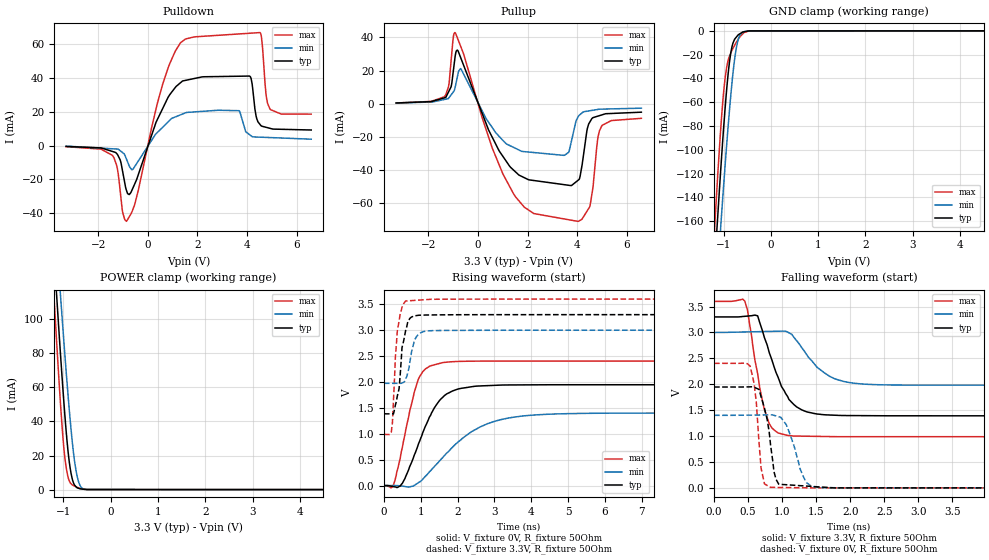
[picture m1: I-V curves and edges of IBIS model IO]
| Texas Instruments Incorporated
| UCD90120A 12-Rail Power Supply Sequencer and Monitor With ACPI Support
[IBIS ver]   4.1
[File name]   ucd90120a.ibs
[File Rev]   1.0
[Date]   02/22/2018
[Source]
| Texas Instruments Incorporated.
| Analog-eLab Design Center, HPA
| 12500 TI Blvd
| Dallas, TX -75243
[Notes]   Revision History:
| Rev 1.0: 02/22/2018
| - Initial version of the model
| - Model based on simulations from Spectre
| - Model not matched to measurements
| - C_comp although listed in numerical order of value are
|   obtained from varying PVT conditions. For PVT conditions for
|   each specific value refer the buffer description under
|   respective [Model]. IBIS model user is responsible for using
|   appropriate C_comp to simulate for Signal Integrity.
| - Warnings regarding combined Non-monotonicity of various models
|   have been reviewed and considered minor and can be ignored.
[Disclaimer]
| This model is designed as an aid for customers of Texas Instruments.
| TI and its licensors and suppliers make no warranties, either expressed
| or implied, with respect to this  model, including the warranties of
| merchantability or fitness for a particular purpose. The model is
| provided solely on an "as is" basis. The entire risk as to its quality
| and performance is with the customer.
| This model is subject to change without notice. Texas Instruments
| Incorporated is not responsible for updating this model.
[Copyright]
(C) Copyright 2018 Texas Instruments Incorporated.All rights reserved.
|  Component UCD90120ARGC 64-pin VQFN - RGC package
|  Part # UCD90120ARGC
[Component]   UCD90120ARGC
[Manufacturer]  TI
[Package]   |64 VQFN - RGC package
|   typ   min   max
R_pkg   0.14489   0.12907   0.17593
L_pkg   2.43477nH   2.15344nH   3.0062nH
C_pkg   0.32891pF   0.27901pF   0.38082pF
[Pin] signal_name   model_name   R_pin   L_pin   C_pin
1   MON1   TERM   0.17593   3.0062nH   0.34764pF
2   MON2   TERM   0.16294   2.76858nH   0.3702pF
3   MON3   TERM   0.15277   2.59361nH   0.35698pF
4   MON4   TERM   0.14559   2.46457nH   0.34579pF
5   MON5   TERM   0.14186   2.40765nH   0.34125pF
6   MON6   TERM   0.14039   2.35478nH   0.31963pF
7   V33DIO1   POWER   0.14074   2.34483nH   0.30672pF
8   DVSS1   GND   0.14225   2.35787nH   0.29065pF
9   RESETN   TERM   0.14058   2.33179nH   0.29142pF
10   TRCK   TERM   0.14103   2.34909nH   0.30499pF
11   GPIO1   TERM   0.14188   2.37826nH   0.31724pF
12   GPIO2   TERM   0.14504   2.4439nH   0.33589pF
13   GPIO3   TERM   0.14847   2.52657nH   0.35271pF
14   GPIO4   TERM   0.15681   2.65682nH   0.35779pF
15   PMBUS_CLK   IO   0.16414   2.78783nH   0.36485pF
16   PMBUS_DATA   IO   0.17538   2.99779nH   0.34751pF
17   FPWM1/GPIO5   TERM   0.16938   2.90166nH   0.3367pF
18   FPWM2/GPIO6   TERM   0.14986   2.5613nH   0.34805pF
19   FPWM3/GPIO7   TERM   0.14143   2.41244nH   0.34137pF
20   FPWM4/GPIO8   TERM   0.1353   2.29867nH   0.33254pF
21   FPWM5/GPIO9   TERM   0.13147   2.23916nH   0.32796pF
22   FPWM6/GPIO10   TERM   0.12964   2.18198nH   0.30393pF
23   FPWM7/GPIO11   TERM   0.12907   2.15795nH   0.29099pF
24   FPWM8/GPIO12   TERM   0.12949   2.15344nH   0.28322pF
25   GPIO13   TERM   0.13079   2.17294nH   0.27901pF
26   DVSS2   GND   0.06676   1.81017nH   0.33013pF
27   PMBUS_ALERT   TERM   0.12948   2.17885nH   0.3095pF
28   PMBUS_CNTRL   TERM   0.13149   2.2241nH   0.32681pF
29   GPIO14   TERM   0.137   2.33822nH   0.34754pF
30   GPIO15   TERM   0.14579   2.47508nH   0.35253pF
31   PWM1/GPI1   TERM   0.15719   2.66944nH   0.36722pF
32   PWM2/GPI2   TERM   0.1721   2.93718nH   0.34634pF
33   GPIO16   TERM   0.16915   2.89043nH   0.33729pF
34   GPIO17   TERM   0.15872   2.69205nH   0.36052pF
35   GPIO18   TERM   0.15067   2.54906nH   0.34862pF
36   TCK/GPIO19   TERM   0.14609   2.45952nH   0.3434pF
37   TDO/GPIO20   TERM   0.14196   2.39583nH   0.33811pF
38   TDI/GPIO21   TERM   0.14095   2.35148nH   0.31582pF
39   TMS/GPIO22   TERM   0.14039   2.32816nH   0.3024pF
40   TRSTN   TERM   0.14076   2.32332nH   0.28408pF
41   PWM4/GPI4   TERM   0.14183   2.33999nH   0.28799pF
42   PWM3/GPI3   TERM   0.14061   2.33098nH   0.30731pF
43   DVSS3   GND   0.07246   1.96818nH   0.36989pF
44   V33DIO2   POWER   0.14089   2.36582nH   0.33463pF
45   V33D   POWER   0.14342   2.43458nH   0.34854pF
46   V33A   POWER   0.14906   2.52365nH   0.35491pF
47   BPCAP   TERM   0.08082   2.24241nH   0.4207pF
48   AVSS2   GND   0.1673   2.86144nH   0.3429pF
49   AVSS1   GND   0.09187   2.63344nH   0.40403pF
50   MON10   TERM   0.16539   2.79716nH   0.38082pF
51   NC1   NC   0.15249   2.57903nH   0.36065pF
52   MON11   TERM   0.14231   2.40327nH   0.34554pF
53   NC2   NC   0.13558   2.30009nH   0.33649pF
54   MON12   TERM   0.13157   2.21003nH   0.30212pF
55   NC3   NC   0.1383   2.2989nH   0.29679pF
56   MON13   TERM   0.13399   2.22211nH   0.29332pF
57   NC4   NC   0.13085   2.17379nH   0.29018pF
58   V33FB   POWER   0.12921   2.15933nH   0.29609pF
59   MON7   TERM   0.12919   2.17545nH   0.30752pF
60   PMBUS_ADDR1   TERM   0.13093   2.21778nH   0.326pF
61   PMBUS_ADDR0   TERM   0.13577   2.32295nH   0.34501pF
62   MON8   TERM   0.14373   2.44842nH   0.35006pF
63   MON9   TERM   0.1549   2.64059nH   0.36782pF
64   AVSS3   GND   0.08619   2.45988nH   0.39062pF
[Model] TERM
Model_type Terminator
C_comp   0  0  0
| variable   typ   min   max
[Voltage Range]   3.30000V  3.00000V  3.60000V
[POWER Clamp Reference]  3.30000V  3.00000V  3.60000V
[GND Clamp Reference]   0.00000V  0.00000V  0.00000V
[Temperature Range]   27   110   -40
| Models and submodels in the file (2): TERM (Terminator), IO (I/O)
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|   IO 3.3V Model
[Model]   IO
Model_type   I/O
|Signals
Vinl =  0.65V
Vinh =  2.85V
Vmeas = 1.475V
Vref = 3.3V
|Rref = 50Ohm
| variable   typ   min   max
|C_comp Output Disabled   (NOM PVT)   (FAST PVT)   (SLOW PVT)
C_comp   1.475pF   1.443pF   1.508pF
|Junction Temperature
[Temperature Range]   27.0   110.0   -40.0
[Voltage range]   3.3V   3.0V   3.6V
[pullup reference]   3.3V   3.0V   3.6V
[power clamp reference]   3.3V   3.0V   3.6V
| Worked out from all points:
|   slope of the pulldown table from 0 to 0.495 V, typ, clamps not added: 25.7 ohm
|   slope of the pullup table from 0 to 0.495 V, typ, clamps not added: 26.7 ohm
|   GND clamp passes 1 mA (typ) near -0.59 V on its own axis
|   POWER clamp passes 1 mA (typ) near -0.70 V on its own axis
|   falling waveform, V_fixture 3.3V, R_fixture 50Ohm: 20-80 % time 340ps typ, 421ps min, 207ps max; typ from 3.3 V to 1.39 V
|   rising waveform, V_fixture 0V, R_fixture 50Ohm: 20-80 % time 708ps typ, 1.32ns min, 449ps max; typ from 0 V to 1.95 V
|   rising waveform, V_fixture 3.3V, R_fixture 50Ohm: 20-80 % time 191ps typ, 179ps min, 136ps max; typ from 1.39 V to 3.3 V
|   falling waveform, V_fixture 0V, R_fixture 50Ohm: 20-80 % time 137ps typ, 200ps min, 87.7ps max; typ from 1.95 V to 0 V
[Pulldown]
|   Voltage   I(typ)   I(min)   I(max)
-3.3V     -501.7uA   -306.3uA   -648.9uA
-1.433V   -3.458mA   -1.887mA   -5.754mA
-867.3mV  -26.36mA   -7.887mA   -44.81mA
-598.8mV  -24.93mA   -13.94mA   -37.54mA
822.5mV   28.76mA    14.15mA    46.26mA
1.862V    39.67mA    19.93mA    64.32mA
3.681V    41.06mA    20.66mA    66.09mA
4.103V    41.15mA    6.486mA    66.49mA
4.526V    12.46mA    4.989mA    66.9mA
4.785V    10.76mA    4.84mA     28.27mA
4.923V    10.23mA    4.76mA     21.76mA
6.59V     9.23mA     3.797mA    18.61mA
[GND Clamp]
|   Voltage   I(typ)   I(min)   I(max)
-3.3V     -1.646A    -1.552A    -1.764A
-1.199V   -203.9mA   -245.2mA   -173.1mA
-1.164V   -181.5mA   -224.8mA   -148.7mA
-1.141V   -167.2mA   -211.4mA   -133.2mA
-1.119V   -153.7mA   -198.7mA   -119mA
-1.055V   -114.3mA   -162mA     -79.87mA
-952.2mV  -57.94mA   -105.5mA   -35.44mA
-847.3mV  -18.71mA   -54.52mA   -18.74mA
-733.4mV  -5.448mA   -15.18mA   -9.859mA
-669.8mV  -2.845mA   -4.95mA    -5.896mA
-590.3mV  -995.3uA   -1.043mA   -2.432mA
6.59V     0A         0A         0A
[Pullup]
|   Voltage   I(typ)   I(min)   I(max)
-3.3V     518.1uA    447.8uA    523.7uA
-1.363V   3.577mA    2.608mA    4.23mA
-1.19V    7.157mA    3.3mA      10.35mA
-932.3mV  27.47mA    9.295mA    42.97mA
-688.4mV  27.43mA    21.03mA    34.24mA
551.3mV   -19.46mA   -13.8mA    -25.62mA
1.43V     -39.88mA   -26.22mA   -54.12mA
3.485V    -48.74mA   -31.03mA   -69.42mA
4.008V    -46.42mA   -8.697mA   -70.8mA
4.508V    -11.06mA   -4.178mA   -62.05mA
4.98V     -6.738mA   -3.186mA   -13.6mA
6.59V     -5.03mA    -2.61mA    -8.729mA
[POWER Clamp]
|   Voltage   I(typ)   I(min)   I(max)
-3.3V     1.126A     1.059A     1.206A
-1.199V   139.3mA    169mA      114.3mA
-1.141V   114.2mA    146mA      86.88mA
-1.055V   77.88mA    112.5mA    48.83mA
-987.2mV  51.21mA    86.79mA    24.19mA
-947.1mV  36.9mA     72.18mA    14.51mA
-835.6mV  9.528mA    35.24mA    3.429mA
-759mV    2.557mA    16.12mA    2.066mA
-698.2mV  955.7uA    6.78mA     1.273mA
-621.5mV  370.3uA    1.374mA    619.3uA
-479.9mV  32.37uA    36uA       50.4uA
6.59V     0A         0A         0A
[Ramp]
R_load = 50
|   typ   min   max
dV/dt_r   1.16808/7.01565e-010  0.840176/1.30988e-009   1.44243/4.42526e-010
dV/dt_f   1.14541/3.06636e-010  0.610549/4.09332e-010   1.56775/2.07614e-010
[Falling Waveform]
V_fixture = 3.3V
V_fixture_min = 3V
V_fixture_max = 3.6V
R_fixture = 50Ohm
C_fixture = 0F
|   Time   V(typ)   V(min)   V(max)
0s        3.3V       3V         3.6V
450ps     3.312V     3.01V      3.608V
490ps     3.316V     3.011V     3.439V
640ps     3.321V     3.015V     2.204V
740ps     2.898V     3.018V     1.506V
850ps     2.466V     3.021V     1.156V
1.08ns    1.763V     3.008V     1.013V
1.61ns    1.412V     2.229V     991.8mV
2.22ns    1.394V     2.002V     987.3mV
14.98ns   1.391V     1.982V     987.1mV
[Rising Waveform]
V_fixture = 0V
V_fixture_min = 0V
V_fixture_max = 0V
R_fixture = 50Ohm
C_fixture = 0F
|   Time   V(typ)   V(min)   V(max)
|   0   1.02929e-009   2.40092e-009   7.786e-010
0s        443.4uV    408uV      455.8uV
270ps     -22.78mV   408uV      36.05mV
500ps     43.66mV    -10.02mV   738.4mV
700ps     368.1mV    -24.22mV   1.442V
940ps     810.1mV    58.93mV    2.065V
1.29ns    1.399V     306.5mV    2.317V
1.6ns     1.706V     544.1mV    2.375V
2.61ns    1.924V     1.131V     2.403V
3.93ns    1.944V     1.354V     2.404V
15ns      1.947V     1.4V       2.404V
[Rising Waveform]
V_fixture = 3.3V
V_fixture_min = 3V
V_fixture_max = 3.6V
R_fixture = 50Ohm
C_fixture = 0F
|   Time   V(typ)   V(min)   V(max)
0s        1.391V     1.982V     987.1mV
200ps     1.385V     1.974V     1.035V
230ps     1.385V     1.974V     1.214V
360ps     1.72V      1.974V     2.965V
410ps     1.867V     1.974V     3.18V
490ps     2.665V     1.981V     3.441V
590ps     2.997V     2.065V     3.564V
830ps     3.277V     2.807V     3.576V
1.17ns    3.293V     2.985V     3.592V
15ns      3.3V       3V         3.6V
[Falling Waveform]
|Gnd
V_fixture = 0V
V_fixture_min = 0V
V_fixture_max = 0V
R_fixture = 50Ohm
C_fixture = 0F
|   Time   V(typ)   V(min)   V(max)
0s        1.947V     1.4V       2.404V
530ps     1.95V      1.404V     2.35V
620ps     1.925V     1.406V     1.653V
690ps     1.759V     1.407V     382.1mV
830ps     822.2mV    1.409V     9.436mV
880ps     310.2mV    1.4V       8.565mV
950ps     70.21mV    1.374V     7.504mV
1.34ns    36.18mV    138mV      1mV
1.54ns    18.19mV    10.09mV    104.5uV
15ns      1.594nV    3.379nV    1.137nV
